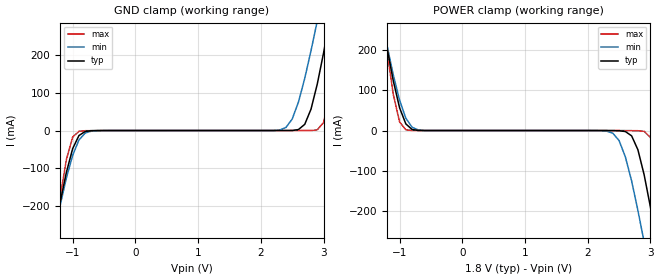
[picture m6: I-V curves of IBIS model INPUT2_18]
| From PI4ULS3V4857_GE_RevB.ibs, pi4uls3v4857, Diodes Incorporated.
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[Model] INPUT2_18
Model_type Input
Vinl = 0.36V
Vinh = 1.44V
| variable   typ   min   max
C_comp   0.809pF   0.803pF   0.816pF
[Voltage Range]   1.8V   1.6V   2.0V
[GND Clamp Reference]   0.000V   0.000V   0.000V
[POWER Clamp Reference]   1.8V   1.6V   2.0V
[temperature range]   40   85   -40
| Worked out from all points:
|   GND clamp passes 1 mA (typ) near -0.73 V on its own axis
|   POWER clamp passes 1 mA (typ) near -0.73 V on its own axis
[GND Clamp]
| Voltage   I(typ)   I(min)   I(max)
-1.8V     -790mA     -723mA     -977mA
-1.3V     -281mA     -277mA     -295mA
-1.1V     -110mA     -125mA     -76.3mA
-1V       -47.6mA    -65.3mA    -17.2mA
-900mV    -13.2mA    -24.9mA    -2.01mA
2.4V      13.3uA     8.07mA     6.71uA
2.7V      16.4mA     138mA      7.85uA
2.9V      123mA      290mA      1.78mA
3V        205mA      374mA      21.4mA
3.1V      297mA      460mA      89.4mA
3.3V      493mA      638mA      321mA
3.6V      805mA      913mA      736mA
[POWER Clamp]   |Note: Vtable = Vcc - Voutput
| Voltage   I(typ)   I(min)   I(max)
-1.8V     805mA      729mA      1.03A
-1.3V     297mA      290mA      321mA
-1V       56.5mA     75.3mA     21.4mA
-900mV    16.4mA     30.5mA     1.78mA
-600mV    13.3uA     113uA      7.27uA
2.4V      -173uA     -6.63mA    -1.22uA
2.7V      -13.2mA    -125mA     -265uA
2.9V      -110mA     -277mA     -2.01mA
3V        -190mA     -362mA     -17.2mA
3.1V      -281mA     -449mA     -76.3mA
3.3V      -477mA     -630mA     -295mA
3.6V      -790mA     -910mA     -696mA
